(* Logix 5000 AddOnInstructionDefinition export NORD_VFDcontrol_XU4_Inst100_101; software revision 24.02 *)

TYPE FI_Data_IN :
STRUCT
   ConnectionFaulted : BOOL;
   RunMode : BOOL;
   Data : INT[6];   // Actual Values
END_STRUCT
END_TYPE

TYPE FI_Data_OUT :
STRUCT
   Data : INT[6];   // Control Data
END_STRUCT
END_TYPE

ADD_ON_INSTRUCTION NORD_VFDcontrol_XU4_Inst100_101   (* revision 1.1, vendor NORD Drivesystems, ExecutePrescan *)
// Control Block for NORD VFD: CU4/TU4
// Revision note:
// Rev 1.1
// Better Ready Start Condition Logic
// Added Inhibited Output
// Added Fault Active Output
// Rev 1.0
// Connection to CU4/TU4-ETH (or EIP)
// Instances: Output 110/Input 111
// For VFD Series:
//    - BASE (SK 180E Series)
//    - FLEX (SK 200E Series)
//    - LINK (SK 250E-FDS Series)
// Allows for control of One VFD only.
//    - No access to remote IO
VAR_IN_OUT
   FI_Status : _0342:CU4_ETH_DE5BFA94:I:0; {required}   // Input Data Map of VFD
   FI_Control : _0342:CU4_ETH_E8E6FFA2:O:0; {required}   // Output Data Map of VFD
END_VAR
VAR_INPUT
   VFD_Number : SINT := 1;   // Number of VFD to control (1 for Instance 100/101)
   EnableFwd : BOOL; {visible}   // HIGH = Enable CW
   EnableRev : BOOL; {visible}   // HIGH = Enable CCW
   DisableVoltage : BOOL := 1; {visible}   // LOW = No Output Voltage
   QuickStop : BOOL := 1; {visible}   // LOW = Emergency Stop Active
   FaultAckn : BOOL; {visible}   // Error / Fault Acknowledgement on Rising Edge
   ParameterSet : SINT := 1; {visible}   // Parameter Set Range 1-4, If less than 1 or greater than 4, set to default of 1
   Activate32BitSetpoint : BOOL; {visible}   // HIGH = Activate 32Bit Setpoint combining Setpoint 2 & 3
   ControlWordBit8_P480_11 : BOOL; {visible}   // Control Word Bit 8 Function set in P480[11]
   ControlWordBit9_P480_12 : BOOL; {visible}   // Control Word Bit 9 Function set in P480[12]
   ControlWord : ALIAS FOR Control_Word; {access None, visible}   // Control Word Read Only Version
   Setpoint1 : INT; {visible}   // Setpoint 1 Function set in P546[1]
   Setpoint2 : INT; {visible}   // Setpoint 2 Function set in P546[2], deactivated if "PositioningActiveBitt" is set
   Setpoint3 : INT; {visible}   // Setpoint 3 Function set in P546[3], deactivated if "PositioningActiveBitt" is set
   Setpoint4 : INT;   // Setpoint 4 Reserved
   Setpoint5 : INT;   // Setpoint 5 Reserved
   Setpoint2_3_32 : DINT; {visible}   // 32 Bit Setpoint 2 & 3 combined for positioning
END_VAR
VAR_OUTPUT
   StatusWord : INT; {access Read Only, visible}   // Status Word
        .0   // Ready to Start
        .1   // Ready for Operation
        .2   // Operation Enabled
        .3   // Fault
        .4   // Voltage Enabled
        .5   // No Emergency Stop
        .6   // Starting Disabled
        .7   // Warning Active
        .8   // Setpoint Reached
        .9   // Bus Controller Active
        .10   // Function P481[9]
        .11   // Rotation Right Active
        .12   // Rotation Left Active
        .13   // Function P481[10]
        .14   // Parameter Set Bit 0
        .15   // Parameter Set Bit 1
   ActiveParameterSet : SINT; {access Read Only, visible}   // Displays active parameter set
   CommunicationOK : BOOL; {access Read Only, visible}   // HIGH = Communication is OK
   ReadyToStart : BOOL; {access Read Only, visible}   // HIGH = Drive Ready to Start
   VFD_Enabled : BOOL; {access Read Only, visible}   // HIGH = VFD is Enabled
   Inhibited : BOOL; {access Read Only, visible}   // VFD is Inhibited
   Warning : BOOL; {access Read Only, visible}   // HIGH = Drive has a Warning
   Faulted : BOOL; {access Read Only, visible}   // HIGH = Drive Faulted
   FaultActive : BOOL; {access Read Only, visible}   // Fault Conditions are Currently Active
   StatusWordBit10_P481_9 : BOOL; {access Read Only, visible}   // Status Word Bit 10 Function set in P481[09]
   StatusWordBit13_P481_10 : BOOL; {access Read Only, visible}   // Status Word Bit 13 Function set in P481[10]
   ActualValue1 : INT; {access Read Only, visible}   // Actual Value 1 Function set in P543[1]
   ActualValue2 : INT; {access Read Only, visible}   // Actual Value 2 Function set in P543[2]
   ActualValue3 : INT; {access Read Only, visible}   // Actual Value 3 Function set in P543[3]
   ActualValue4 : INT; {access Read Only}   // Actual Value 4 Reserved
   ActualValue5 : INT; {access Read Only}   // Actual Value 5 Reserved
   ActualValue2_3_32 : DINT; {access Read Only, visible}   // 32 Bit Actual Value 2 & 3 Combined for Positioning
END_VAR
VAR
   Index : INT; {access None}   // Index of process data based on VFD_Number
   Control_Word : INT; {access None}   // Control Word
        .0   // Enable Operation
        .1   // Disable Voltage (Low level disables the output voltage of the drive and stops the VFD)
        .2   // Emergency Stop (Low level activates QuickStop mode and stops the VFD)
        .3   // Ready for Operation
        .4   // Enable Pulses
        .5   // Enable Ramp
        .6   // Enable Setpoint
        .7   // Error Acknowledge
        .8   // Function P480[11]
        .9   // Function P480[12]
        .10   // Control Data Valid
        .11   // Rotation Direction Clockwise
        .12   // Rotation Direction Counter-Clockwise
        .13   // Reserved
        .14   // Parameter Set Bit 0
        .15   // Parameter Set Bit 1
   Control : FI_Data_OUT; {access None}
   Status : FI_Data_IN; {access None}
   LowWordOf32BitSetpoint : DINT; {access None}
   Temporary_Variable_32BitSepoint : DINT; {access None}
   HighWordOf32BitSetpoint : DINT; {access None}
END_VAR

ROUTINE Logic   (* ladder *)
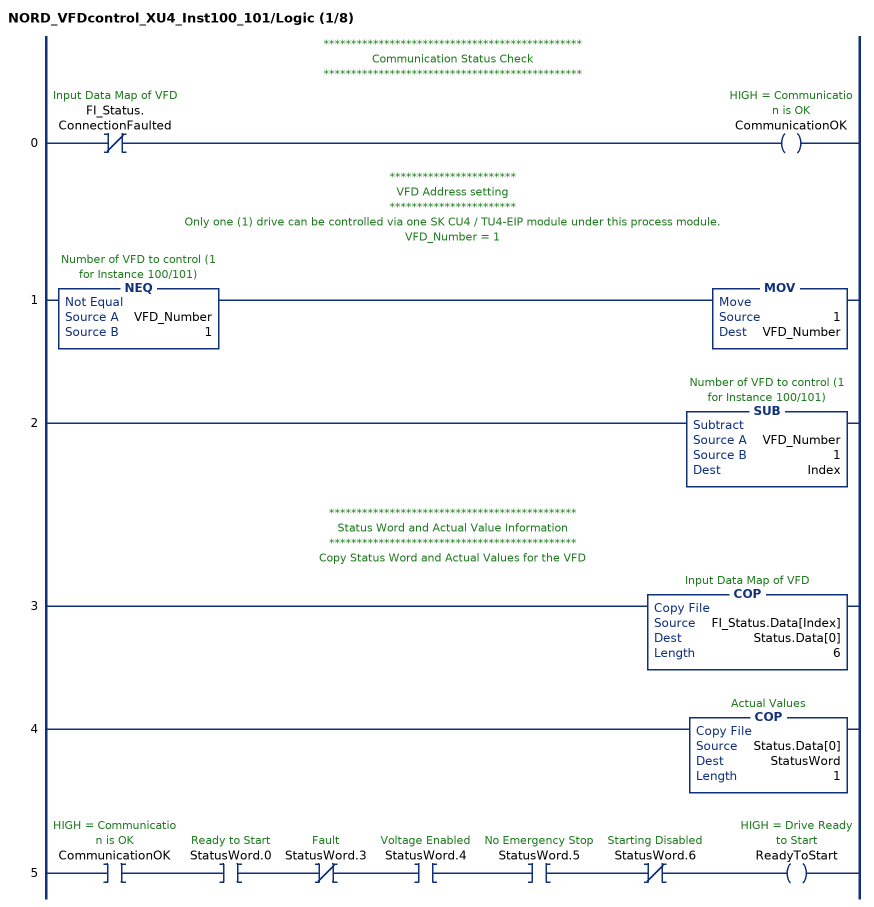
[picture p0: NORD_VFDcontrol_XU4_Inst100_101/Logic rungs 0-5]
   // ***********************************************
   // Communication Status Check
   // ***********************************************
   0: XIO(FI_Status.ConnectionFaulted)OTE(CommunicationOK);
   // ***********************
   // VFD Address setting
   // ***********************
   // Only one (1) drive can be controlled via one SK CU4 / TU4-EIP module under this process module.
   // VFD_Number = 1
   1: NEQ(VFD_Number,1)MOV(1,VFD_Number);
   2: SUB(VFD_Number,1,Index);
   // *********************************************
   // Status Word and Actual Value Information
   // *********************************************
   // Copy Status Word and Actual Values for the VFD
   3: COP(FI_Status.Data[Index],Status.Data[0],6);
   4: COP(Status.Data[0],StatusWord,1);
   5: XIC(CommunicationOK)XIC(StatusWord.0)XIO(StatusWord.3)XIC(StatusWord.4)XIC(StatusWord.5)XIO(StatusWord.6)OTE(ReadyToStart);
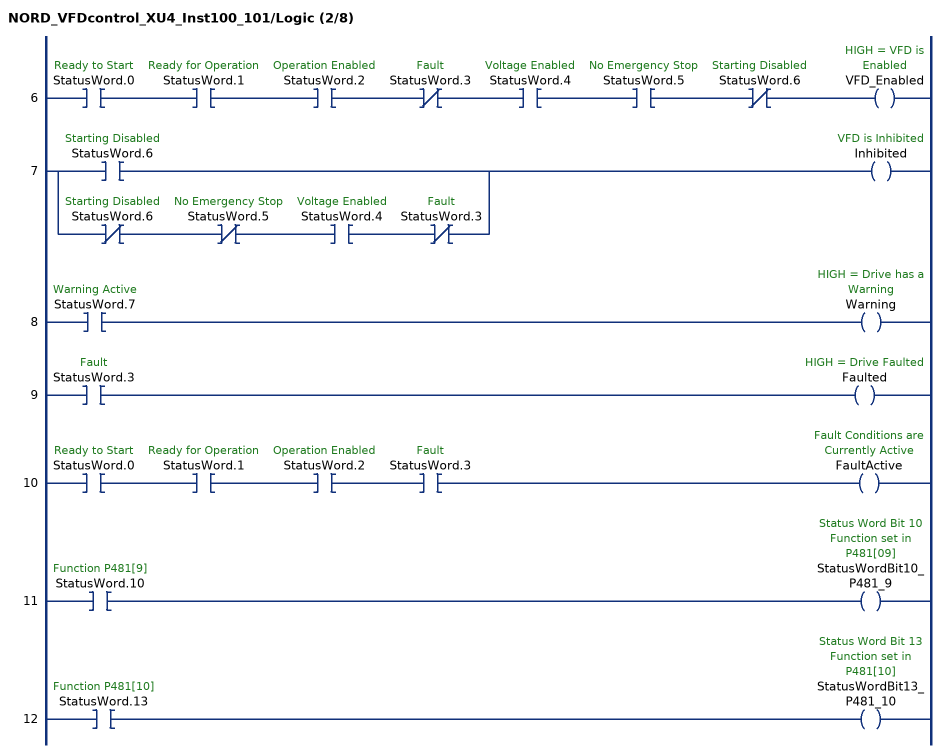
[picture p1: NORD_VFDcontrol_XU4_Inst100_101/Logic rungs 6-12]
   6: XIC(StatusWord.0)XIC(StatusWord.1)XIC(StatusWord.2)XIO(StatusWord.3)XIC(StatusWord.4)XIC(StatusWord.5)XIO(StatusWord.6)OTE(VFD_Enabled);
   7: [XIC(StatusWord.6) ,XIO(StatusWord.6) XIO(StatusWord.5) XIC(StatusWord.4) XIO(StatusWord.3) ]OTE(Inhibited);
   8: XIC(StatusWord.7)OTE(Warning);
   9: XIC(StatusWord.3)OTE(Faulted);
   10: XIC(StatusWord.0)XIC(StatusWord.1)XIC(StatusWord.2)XIC(StatusWord.3)OTE(FaultActive);
   11: XIC(StatusWord.10)OTE(StatusWordBit10_P481_9);
   12: XIC(StatusWord.13)OTE(StatusWordBit13_P481_10);
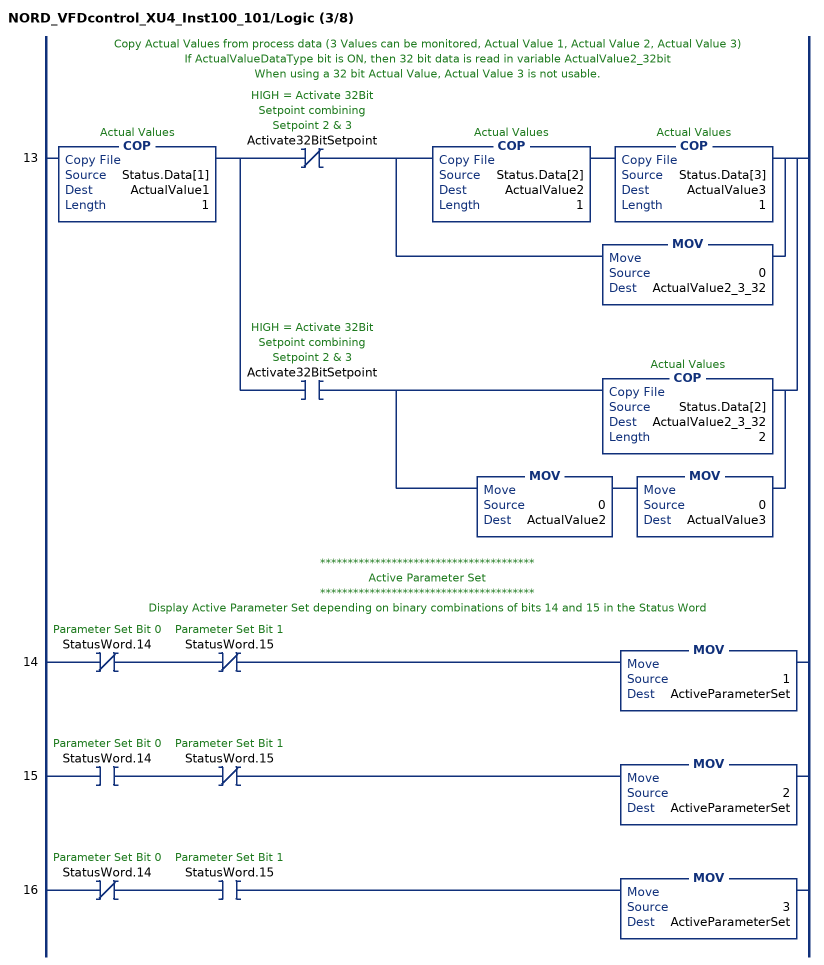
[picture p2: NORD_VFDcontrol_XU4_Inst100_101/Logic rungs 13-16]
   // Copy Actual Values from process data (3 Values can be monitored, Actual Value 1, Actual Value 2, Actual Value 3)
   // If ActualValueDataType bit is ON, then 32 bit data is read in variable ActualValue2_32bit
   // When using a 32 bit Actual Value, Actual Value 3 is not usable.
   13: COP(Status.Data[1],ActualValue1,1)[XIO(Activate32BitSetpoint) [COP(Status.Data[2],ActualValue2,1) COP(Status.Data[3],ActualValue3,1) ,MOV(0,ActualValue2_3_32) ] ,XIC(Activate32BitSetpoint) [COP(Status.Data[2],ActualValue2_3_32,2) ,MOV(0,ActualValue2) MOV(0,ActualValue3) ] ];
   // ***************************************
   // Active Parameter Set
   // ***************************************
   // Display Active Parameter Set depending on binary combinations of bits 14 and 15 in the Status Word
   14: XIO(StatusWord.14)XIO(StatusWord.15)MOV(1,ActiveParameterSet);
   15: XIC(StatusWord.14)XIO(StatusWord.15)MOV(2,ActiveParameterSet);
   16: XIO(StatusWord.14)XIC(StatusWord.15)MOV(3,ActiveParameterSet);
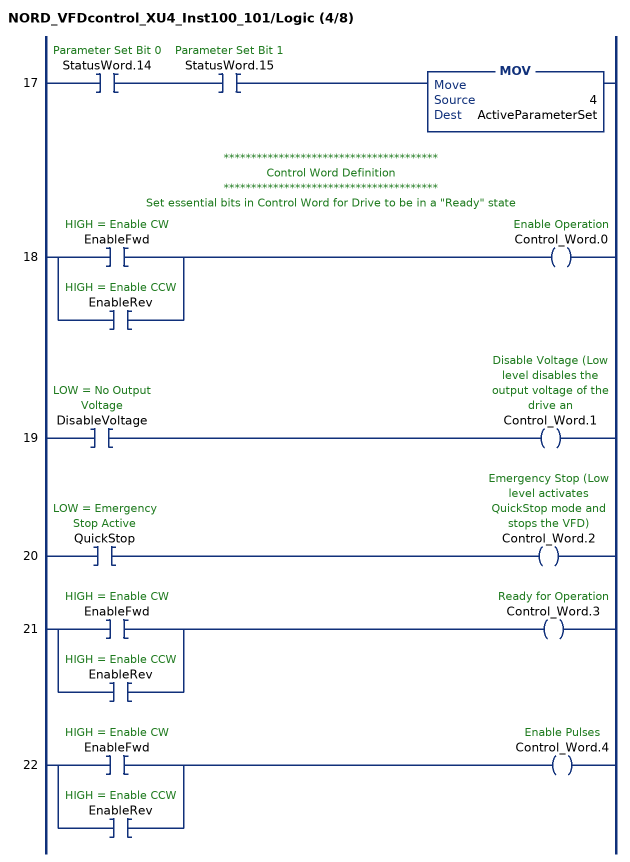
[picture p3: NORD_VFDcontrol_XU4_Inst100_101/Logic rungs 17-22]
   17: XIC(StatusWord.14)XIC(StatusWord.15)MOV(4,ActiveParameterSet);
   // ***************************************
   // Control Word Definition
   // ***************************************
   // Set essential bits in Control Word for Drive to be in a "Ready" state
   18: [XIC(EnableFwd) ,XIC(EnableRev) ]OTE(Control_Word.0);
   19: XIC(DisableVoltage)OTE(Control_Word.1);
   20: XIC(QuickStop)OTE(Control_Word.2);
   21: [XIC(EnableFwd) ,XIC(EnableRev) ]OTE(Control_Word.3);
   22: [XIC(EnableFwd) ,XIC(EnableRev) ]OTE(Control_Word.4);
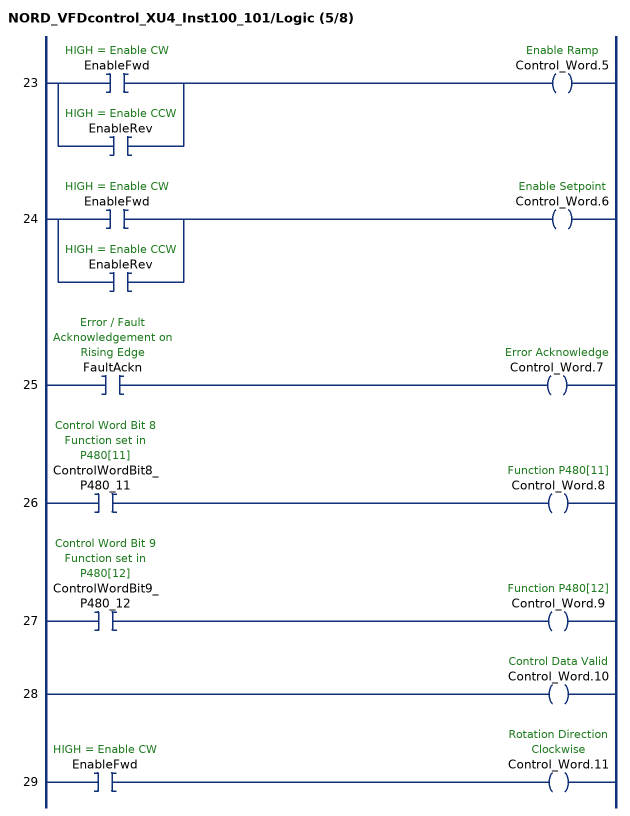
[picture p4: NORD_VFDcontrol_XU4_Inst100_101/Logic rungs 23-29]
   23: [XIC(EnableFwd) ,XIC(EnableRev) ]OTE(Control_Word.5);
   24: [XIC(EnableFwd) ,XIC(EnableRev) ]OTE(Control_Word.6);
   25: XIC(FaultAckn)OTE(Control_Word.7);
   26: XIC(ControlWordBit8_P480_11)OTE(Control_Word.8);
   27: XIC(ControlWordBit9_P480_12)OTE(Control_Word.9);
   28: OTE(Control_Word.10);
   29: XIC(EnableFwd)OTE(Control_Word.11);
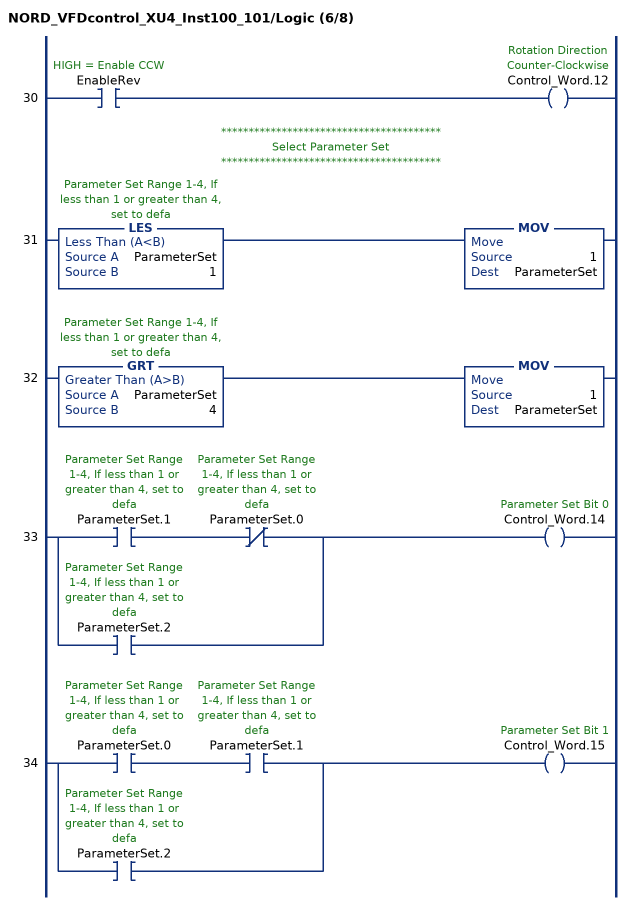
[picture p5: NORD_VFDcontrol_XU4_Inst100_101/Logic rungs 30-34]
   30: XIC(EnableRev)OTE(Control_Word.12);
   // ****************************************
   // Select Parameter Set
   // ****************************************
   31: LES(ParameterSet,1)MOV(1,ParameterSet);
   32: GRT(ParameterSet,4)MOV(1,ParameterSet);
   33: [XIC(ParameterSet.1) XIO(ParameterSet.0) ,XIC(ParameterSet.2) ]OTE(Control_Word.14);
   34: [XIC(ParameterSet.0) XIC(ParameterSet.1) ,XIC(ParameterSet.2) ]OTE(Control_Word.15);
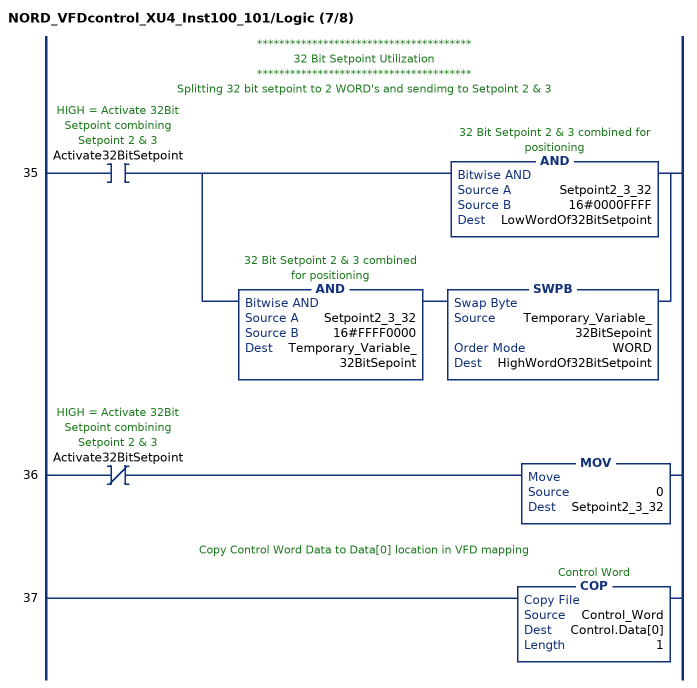
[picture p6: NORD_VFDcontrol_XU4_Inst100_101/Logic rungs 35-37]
   // ***************************************
   // 32 Bit Setpoint Utilization
   // ***************************************
   // Splitting 32 bit setpoint to 2 WORD's and sendimg to Setpoint 2 & 3
   35: XIC(Activate32BitSetpoint)[AND(Setpoint2_3_32,16#0000FFFF,LowWordOf32BitSetpoint) ,AND(Setpoint2_3_32,16#FFFF0000,Temporary_Variable_32BitSepoint) SWPB(Temporary_Variable_32BitSepoint,WORD,HighWordOf32BitSetpoint) ];
   36: XIO(Activate32BitSetpoint)MOV(0,Setpoint2_3_32);
   // Copy Control Word Data to Data[0] location in VFD mapping
   37: COP(Control_Word,Control.Data[0],1);
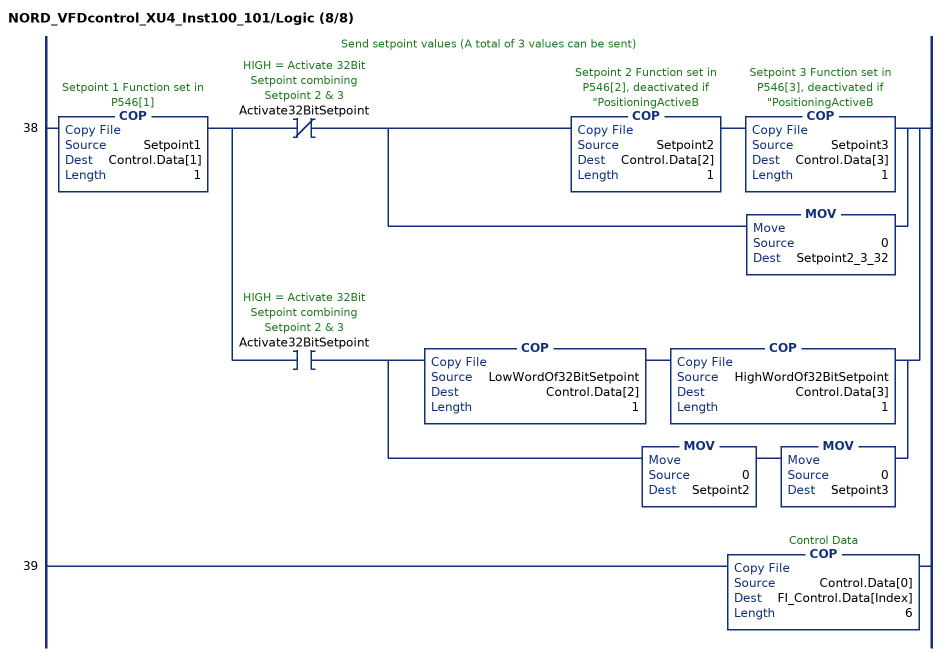
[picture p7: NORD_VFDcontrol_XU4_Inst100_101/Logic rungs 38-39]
   // Send setpoint values (A total of 3 values can be sent)
   38: COP(Setpoint1,Control.Data[1],1)[XIO(Activate32BitSetpoint) [COP(Setpoint2,Control.Data[2],1) COP(Setpoint3,Control.Data[3],1) ,MOV(0,Setpoint2_3_32) ] ,XIC(Activate32BitSetpoint) [COP(LowWordOf32BitSetpoint,Control.Data[2],1) COP(HighWordOf32BitSetpoint,Control.Data[3],1) ,MOV(0,Setpoint2) MOV(0,Setpoint3) ] ];
   39: COP(Control.Data[0],FI_Control.Data[Index],6);
END_ROUTINE

ROUTINE Prescan   (* ladder *)
// Executed prior to first scan of AOI
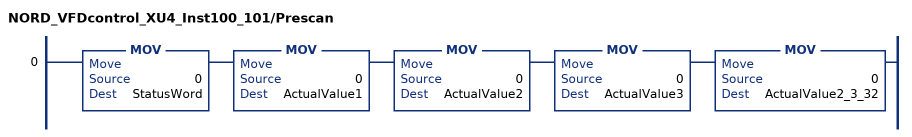
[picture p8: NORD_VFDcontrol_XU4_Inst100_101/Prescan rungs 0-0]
   0: MOV(0,StatusWord)MOV(0,ActualValue1)MOV(0,ActualValue2)MOV(0,ActualValue3)MOV(0,ActualValue2_3_32);
END_ROUTINE
END_ADD_ON_INSTRUCTION
